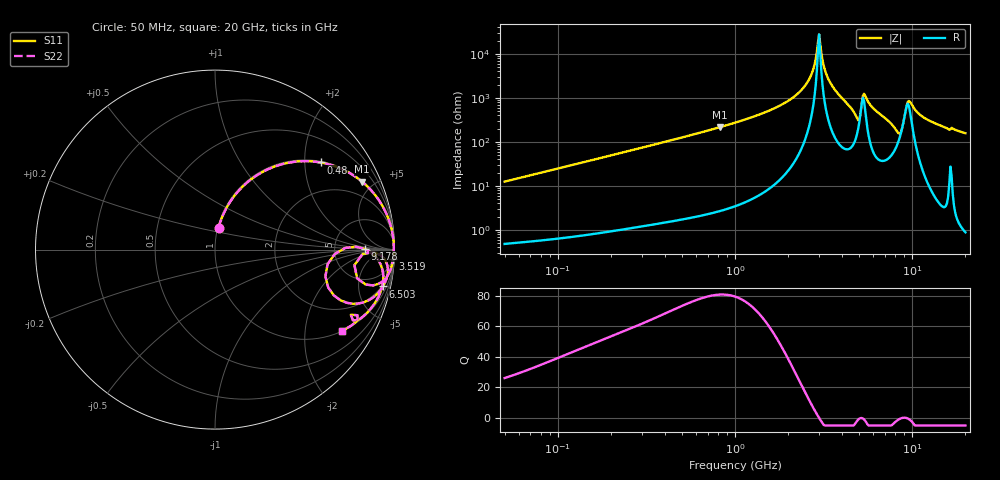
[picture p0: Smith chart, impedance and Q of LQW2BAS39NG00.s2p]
!Murata Part Number: LQW2BAS39NG00
!These Parameters are Measured in Series Mode Connection
!  o--[Z]--o
!Port1  Port2
!  o-------o
!Freq. Start=50[MHz] Stop=20[GHz], 401[Steps]
# Hz S RI R 50
!Freq.(Hz) S11(Real) S11(Imag) S21(Real) S21(Imag) S12(Real) S12(Imag) S22(Real) S22(Imag)
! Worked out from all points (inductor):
!   401 points, 50 MHz to 20 GHz, reference 50 ohm
!   read as one part in series: L = 39.4 nH near 51.52 MHz
!   highest Q = 80.8 at 823.1 MHz (marker M1), where L = 41.7 nH
!   self-resonance near 2.94 GHz
!   S11 on the Smith chart (normalised r, x): 50 MHz: 1.01, +0.25; 480 MHz: 1.03, +2.40; 3.519 GHz: 5, -38; 6.503 GHz: 1.78, -8.88; 9.178 GHz: 11, +0; 20 GHz: 1.02, -3.14
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5e7  0.0197 0.1212  0.9803 -0.1212  0.9803 -0.1212  0.0197 0.1212
1.364002e8  0.1067 0.298  0.8933 -0.298  0.8933 -0.298  0.1067 0.298
3.721004e8  0.4596 0.4909  0.5404 -0.4909  0.5404 -0.4909  0.4596 0.4909
4.800071e8  0.5882 0.4853  0.4118 -0.4853  0.4118 -0.4853  0.5882 0.4853
8.230629e8  0.8197 0.3783  0.1803 -0.3783  0.1803 -0.3783  0.8197 0.3783
1e9  0.8777 0.3214  0.1223 -0.3214  0.1223 -0.3214  0.8777 0.3214
2.021818e9  0.9844 0.1112  0.0156 -0.1112  0.0156 -0.1112  0.9844 0.1112
2.419936e9  0.9933 0.0602  0.00674 -0.0602  0.00674 -0.0602  0.9933 0.0602
2.728004e9  0.996 0.026  0.00399 -0.026  0.00399 -0.026  0.996 0.026
2.98453e9  0.9964 -0.000128  0.00361 0.000128  0.00361 0.000128  0.9964 -0.000128
3.265178e9  0.9952 -0.0272  0.00485 0.0272  0.00485 0.0272  0.9952 -0.0272
3.519108e9  0.9926 -0.0509  0.00741 0.0509  0.00741 0.0509  0.9926 -0.0509
4.89267e9  0.8389 -0.1947  0.1611 0.1947  0.1611 0.1947  0.8389 -0.1947
5.433528e9  0.9552 -0.0727  0.0448 0.0727  0.0448 0.0727  0.9552 -0.0727
6.503449e9  0.9358 -0.2052  0.0642 0.2052  0.0642 0.2052  0.9358 -0.2052
7.442007e9  0.8561 -0.2819  0.1439 0.2819  0.1439 0.2819  0.8561 -0.2819
8.020766e9  0.7367 -0.2969  0.2633 0.2969  0.2633 0.2969  0.7367 -0.2969
8.516016e9  0.6152 -0.1497  0.3848 0.1497  0.3848 0.1497  0.6152 -0.1497
9.178299e9  0.833 0.00503  0.167 -0.00503  0.167 -0.00503  0.833 0.00503
9.745021e9  0.9246 -0.087  0.0754 0.087  0.0754 0.087  0.9246 -0.087
1.220001e10  0.9022 -0.2791  0.0978 0.2791  0.0978 0.2791  0.9022 -0.2791
2e10  0.7097 -0.4511  0.2903 0.4511  0.2903 0.4511  0.7097 -0.4511
